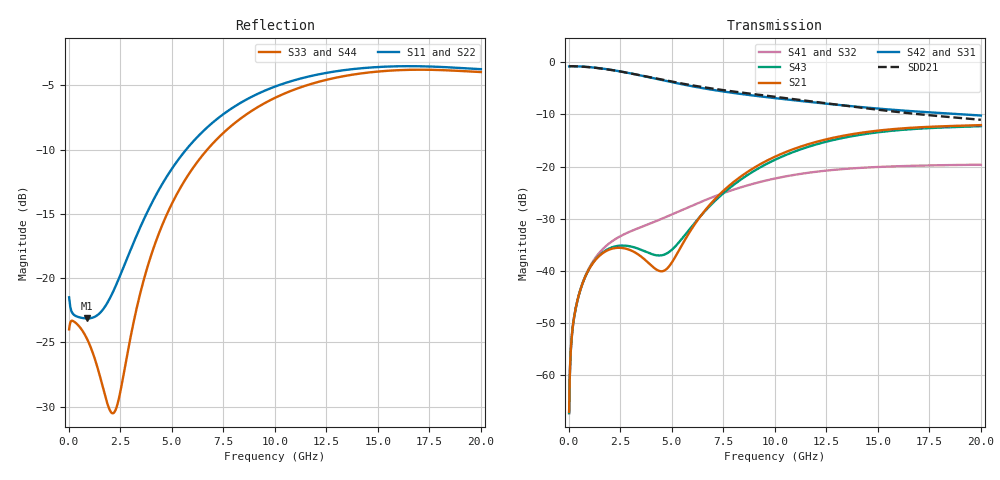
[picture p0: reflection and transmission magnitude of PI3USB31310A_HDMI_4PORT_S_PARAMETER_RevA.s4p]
! NPort=4 DATA=800 NOISE=0 GROUPDELAY=0 COMPLEX_DATAFORMAT=POLAR
! NumOfBlock=1 NumOfParam=0
! .MODEL Smodel S TSTONEFILE=PI3USB31310A_HDMI_4PORT_S_PARAMETER_RevA.s4p TYPE=S
!  -- The above .MODEL line can be used for the S element in the netlist.
!  Port definition:
!  Port1 = INPUT+
!  Port2 = INPUT-
!  Port3 = OUTPUT+
!  Port4 = OUTPUT-
# Hz S MA R  50
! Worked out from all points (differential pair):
!   800 points, 25 MHz to 20 GHz, reference 50 ohm
!   strongest paths, dB at 25 MHz, 5.025 GHz, 10.03 GHz, 15.03 GHz, 20 GHz:
!     S42: -0.8, -3.8, -6.9, -8.9, -10.2
!     S31: -0.8, -3.8, -6.9, -8.9, -10.2
!     S21: -67.0, -38.3, -18.1, -13.1, -12.1
!     S43: -67.2, -35.9, -18.7, -13.4, -12.3
!     S41: -67.2, -29.1, -22.3, -20.1, -19.6
!     S32: -67.2, -29.1, -22.3, -20.1, -19.6
!   taken as a pair (ports 2,1 in; 4,3 out), SDD21 dB: -0.8, -3.7, -6.6, -9.1, -11.0
!   lowest |S11| = -23.1 dB at 900 MHz (marker M1), VSWR 1.15, Z = 53.6 - j6.29 ohm
!   |S11| at or under -10 dB: start of sweep to 5.698 GHz
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2.5e7  0.08424 -5.6  0.0004476 86.3  0.9312 -0.8  0.0004437 86.3
       0.0004476 86.3  0.08424 -5.6  0.0004437 86.3  0.9312 -0.8
       0.9103 -0.3  0.0004341 86.8  0.0632 1.5  0.0004366 86.9
       0.0004341 86.8  0.9103 -0.3  0.0004366 86.9  0.0632 1.5
2.75e8  0.07183 -19.7  0.003706 71.3  0.9169 -4.9  0.003684 71.0
        0.003706 71.3  0.07183 -19.7  0.003684 71.0  0.9169 -4.9
        0.9144 -4.6  0.003674 71.3  0.06767 -9.2  0.003694 72.1
        0.003674 71.3  0.9144 -4.6  0.003694 72.1  0.06767 -9.2
9e8  0.06969 -56.9  0.009647 66.6  0.9018 -15.1  0.009818 65.7
     0.009647 66.6  0.06969 -56.9  0.009818 65.7  0.9018 -15.1
     0.9003 -15.1  0.009802 65.8  0.0579 -33.4  0.009662 68.3
     0.009802 65.8  0.9003 -15.1  0.009662 68.3  0.0579 -33.4
2.225e9  0.09099 -144.1  0.01656 50.7  0.8352 -35.9  0.02 48.7
         0.01656 50.7  0.09099 -144.1  0.02 48.7  0.8352 -35.9
         0.8339 -35.9  0.01997 48.7  0.03012 -135.2  0.01715 55.2
         0.01997 48.7  0.8339 -35.9  0.01715 55.2  0.03012 -135.2
4.65e9  0.2403 119.9  0.01011 91.2  0.6671 -67.0  0.03251 32.4
        0.01011 91.2  0.2403 119.9  0.03251 32.4  0.6671 -67.0
        0.6661 -67.0  0.03245 32.5  0.1687 103.4  0.01439 85.5
        0.03245 32.5  0.6661 -67.0  0.01439 85.5  0.1687 103.4
7.625e9  0.4417 56.3  0.06154 130.2  0.5203 -94.9  0.05684 8.8
         0.06154 130.2  0.4417 56.3  0.05684 8.8  0.5203 -94.9
         0.5194 -94.9  0.05675 8.8  0.375 49.3  0.05819 122.2
         0.05675 8.8  0.5194 -94.9  0.05819 122.2  0.375 49.3
2e10  0.6507 -56.6  0.2496 45.1  0.3089 153.8  0.1043 -141.3
      0.2496 45.1  0.6507 -56.6  0.1043 -141.3  0.3089 153.8
      0.3084 153.8  0.1042 -141.3  0.6341 -57.2  0.2438 45.5
      0.1042 -141.3  0.3084 153.8  0.2438 45.5  0.6341 -57.2
